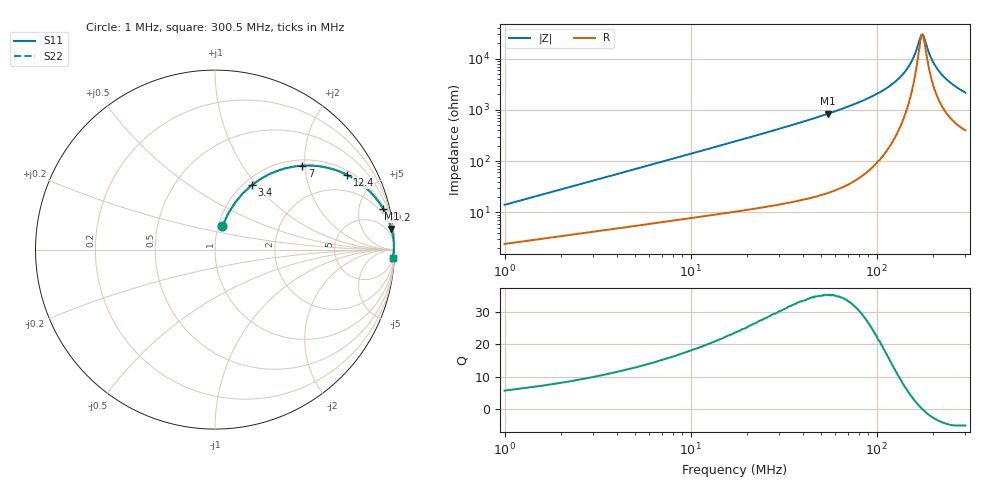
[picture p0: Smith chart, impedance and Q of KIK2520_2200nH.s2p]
!version-2
!date-01.2022
!Series
# MHz S RI R 50
!Freq ReS11 ImS11 ReS21 ImS21 ReS12 ImS12 ReS22 ImS22
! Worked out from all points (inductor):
!   500 points, 1 MHz to 300.5 MHz, reference 50 ohm
!   read as one part in series: L = 2.2 uH near 2.2 MHz
!   highest Q = 35.1 at 55 MHz (marker M1), where L = 2.44 uH
!   self-resonance near 176.5 MHz
!   S11 on the Smith chart (normalised r, x): 1 MHz: 1.05, +0.28; 3.4 MHz: 1.09, +0.94; 7 MHz: 1.13, +1.94; 12.4 MHz: 1.17, +3.45; 29.2 MHz: 1.28, +8.30; 300.5 MHz: 9, -43
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1  0.0411 0.1294  0.9589 -0.1294  0.9589 -0.1294  0.0411 0.1294
3.4  0.204 0.3583  0.796 -0.3583  0.796 -0.3583  0.204 0.3583
5.2  0.3531 0.441  0.6469 -0.441  0.6469 -0.441  0.3531 0.441
7  0.4863 0.4678  0.5137 -0.4678  0.5137 -0.4678  0.4863 0.4678
9.4  0.6233 0.4568  0.3767 -0.4568  0.3767 -0.4568  0.6233 0.4568
12.4  0.7381 0.4154  0.2619 -0.4154  0.2619 -0.4154  0.7381 0.4154
19  0.8663 0.3206  0.1337 -0.3206  0.1337 -0.3206  0.8663 0.3206
29.2  0.9385 0.224  0.0615 -0.224  0.0615 -0.224  0.9385 0.224
51.4  0.9802 0.1256  0.0198 -0.1256  0.0198 -0.1256  0.9802 0.1256
55  0.9829 0.1162  0.0171 -0.1162  0.0171 -0.1162  0.9829 0.1162
101  0.9956 0.0475  0.00445 -0.0475  0.00445 -0.0475  0.9956 0.0475
131  0.997 0.0248  0.00302 -0.0248  0.00302 -0.0248  0.997 0.0248
151  0.9971 0.0126  0.00292 -0.0126  0.00292 -0.0126  0.9971 0.0126
161  0.997 0.00756  0.00303 -0.00756  0.00303 -0.00756  0.997 0.00756
172  0.9967 0.00198  0.00326 -0.00198  0.00326 -0.00198  0.9967 0.00198
176  0.9966 0.000295  0.00335 -0.000295  0.00335 -0.000295  0.9966 0.000295
179  0.9966 -0.00108  0.00344 0.00108  0.00344 0.00108  0.9966 -0.00108
190  0.9962 -0.00609  0.00381 0.00609  0.00381 0.00609  0.9962 -0.00609
201  0.9958 -0.0106  0.00423 0.0106  0.00423 0.0106  0.9958 -0.0106
223  0.9947 -0.0192  0.00526 0.0192  0.00526 0.0192  0.9947 -0.0192
251  0.9932 -0.0288  0.00684 0.0288  0.00684 0.0288  0.9932 -0.0288
300.5  0.9897 -0.0443  0.0103 0.0443  0.0103 0.0443  0.9897 -0.0443
